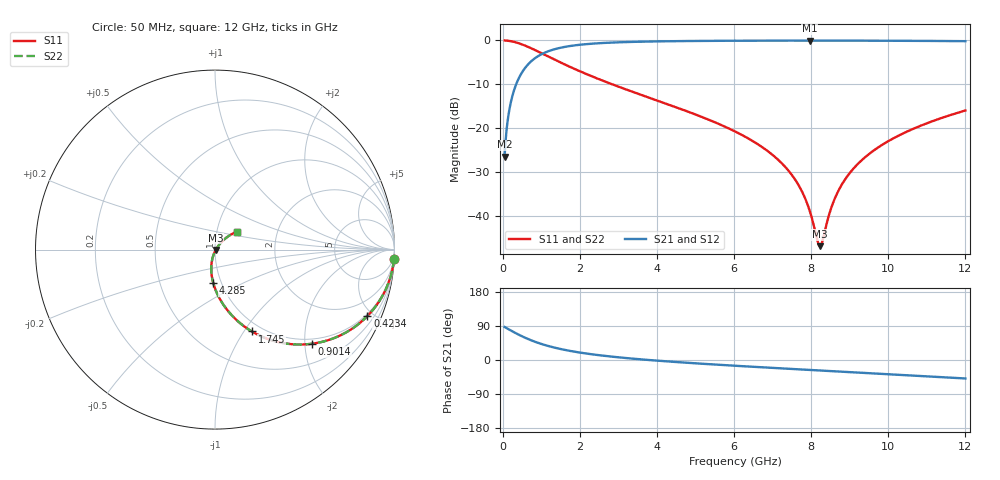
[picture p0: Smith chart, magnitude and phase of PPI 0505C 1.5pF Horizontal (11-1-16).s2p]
# MHz S MA R 50
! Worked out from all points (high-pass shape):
!   1601 points, 50 MHz to 12 GHz, reference 50 ohm
!   highest |S21| = -0.04 dB at 7.959 GHz (marker M1); lowest = -26.4 dB at 50 MHz (marker M2)
!   |S21| within 3 dB of the highest: 1.028 GHz to end of sweep
!   lowest |S11| = -46.7 dB at 8.228 GHz (marker M3), VSWR 1.01, Z = 50.4 - j0.221 ohm
!   |S11| at or under -10 dB: 2.849 GHz to end of sweep
!   |S22| runs from -46.7 to 0.0 dB; largest |S21 - S12| = 0
!   S11 on the Smith chart (normalised r, x): 50 MHz: 1, -39; 423.4 MHz: 0.89, -4.64; 901.4 MHz: 0.89, -2.16; 1.745 GHz: 0.89, -1.09; 4.285 GHz: 0.92, -0.36; 12 GHz: 1.25, +0.26
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50  0.9989 -2.9  0.04777 87.1  0.04777 87.1  0.9989 -2.9
147.0938  0.9902 -8.5  0.1393 81.5  0.1393 81.5  0.9902 -8.5
206.8438  0.9809 -11.9  0.1941 78.1  0.1941 78.1  0.9809 -11.9
423.4375  0.9264 -23.5  0.3759 66.4  0.3759 66.4  0.9264 -23.5
901.4375  0.7539 -44.1  0.6556 45.8  0.6556 45.8  0.7539 -44.1
1745.406  0.5005 -65.7  0.8636 24.0  0.8636 24.0  0.5005 -65.7
2044.156  0.438 -70.7  0.8966 19.0  0.8966 19.0  0.438 -70.7
4038.312  0.2052 -91.1  0.9753 -2.0  0.9753 -2.0  0.2052 -91.1
4284.781  0.1879 -92.8  0.9787 -3.8  0.9787 -3.8  0.1879 -92.8
6025  0.09249 -102.8  0.9915 -15.2  0.9915 -15.2  0.09249 -102.8
7294.688  0.0379 -106.0  0.9946 -22.5  0.9946 -22.5  0.0379 -106.0
7683.062  0.02233 -103.3  0.9949 -24.7  0.9949 -24.7  0.02233 -103.3
7959.406  0.0117 -93.6  0.9949 -26.2  0.9949 -26.2  0.0117 -93.6
8019.156  0.009552 -88.3  0.9949 -26.5  0.9949 -26.5  0.009552 -88.3
8161.062  0.005336 -58.3  0.9949 -27.3  0.9949 -27.3  0.005336 -58.3
8228.281  0.004599 -28.5  0.9949 -27.7  0.9949 -27.7  0.004599 -28.5
8295.5  0.00531 1.4  0.9949 -28.0  0.9949 -28.0  0.00531 1.4
8571.844  0.01442 41.3  0.9946 -29.6  0.9946 -29.6  0.01442 41.3
8870.594  0.02601 48.0  0.9943 -31.2  0.9943 -31.2  0.02601 48.0
9348.594  0.04507 49.7  0.9934 -33.8  0.9934 -33.8  0.04507 49.7
10013.31  0.07225 48.3  0.9915 -37.5  0.9915 -37.5  0.07225 48.3
12000  0.1599 39.0  0.9802 -48.8  0.9802 -48.8  0.1599 39.0
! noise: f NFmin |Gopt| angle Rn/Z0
50  0.000954  0.9581  1.695  0.005127
1372  0.005538  0.7567  6.409  0.004589
2701  0.008675  0.7024  10.56  0.005667
4031  0.01144  0.6705  14.76  0.006572
5360  0.01404  0.6495  18.93  0.007411
6682  0.01656  0.6356  23.01  0.008234
8012  0.01909  0.6269  27.03  0.009089
9341  0.02168  0.6223  30.96  0.01
1.067e+04  0.02437  0.6214  34.77  0.011
1.2e+04  0.0272  0.6236  38.49  0.01212
